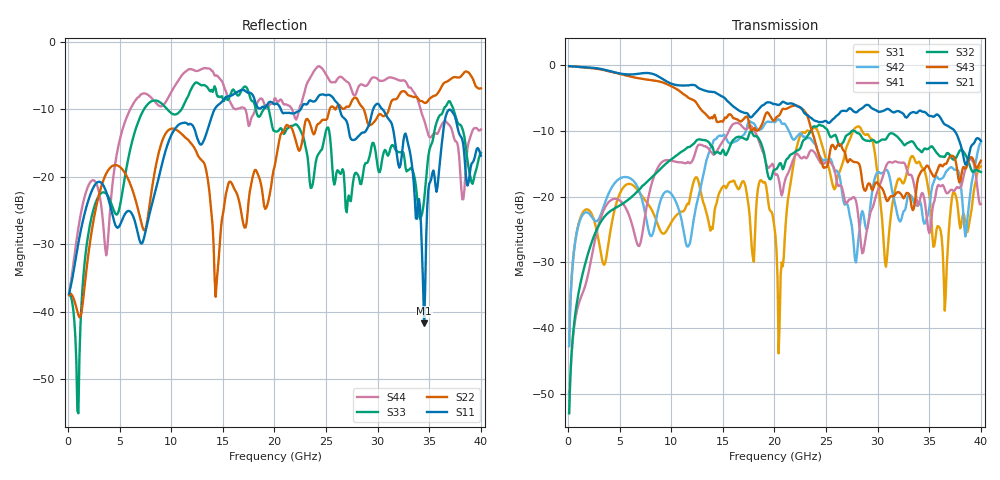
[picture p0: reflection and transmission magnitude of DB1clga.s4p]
! ADC12DJ3200QML-SP
! 196-pin ZMX package
! CLGA Ceramic Package without columns (ceramic land grid array)
! Texas Instruments 4/21/2021
! Single-ended  S-parameters
! PORT#  PORT_NAME  NET_NAME
! PORT1:  DAxN.DIEBUMP DAxN
! PORT2:  DAxN.BGA  DAxN
! PORT3:  DAxP.DIEBUMP DAxP
! PORT4:  DAxP.BGA  DAxP
! Touchstone Ver. 1.0
! Number of ports is 4
# Hz	S	MA	R	50.000000
! SCATTERING PARAMETERS  :
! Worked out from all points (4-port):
!   400 points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, 100 MHz to 40 GHz, reference 50 ohm
!   strongest paths, dB at 100 MHz, 10.1 GHz, 20.1 GHz, 30.1 GHz, 40 GHz:
!     S21: -0.1, -2.8, -5.9, -7.1, -11.5
!     S43: -0.1, -3.2, -8.1, -18.2, -14.5
!     S32: -53.0, -14.2, -15.9, -11.6, -16.2
!     S41: -52.9, -14.5, -16.7, -18.7, -21.1
!     S42: -42.7, -19.8, -8.6, -16.2, -11.7
!     S31: -42.7, -23.6, -26.1, -18.4, -15.3
!   lowest |S11| = -41.7 dB at 34.5 GHz (marker M1), VSWR 1.02, Z = 50.7 + j0.457 ohm
!   |S11| at or under -10 dB: start of sweep to 14.2 GHz; 26.32 GHz to 29.57 GHz (3.243 GHz wide, 11.6 % of centre); 30.45 GHz to end of sweep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
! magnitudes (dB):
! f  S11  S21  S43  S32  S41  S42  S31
! 100 MHz  -37.3  -0.1  -0.1  -53.0  -52.9  -42.7  -42.7
! 4 GHz  -23.8  -0.9  -0.9  -22.3  -20.7  -19.3  -26.2
! 19.1 GHz  -9.8  -5.8  -7.6  -14.3  -14.4  -8.8  -17.8
! 20.4 GHz  -9.4  -6.0  -7.7  -15.2  -17.2  -8.2  -43.8
! 25.3 GHz  -7.9  -8.8  -13.9  -10.6  -14.6  -14.3  -15.8
! 34.5 GHz  -41.7  -7.1  -15.9  -12.7  -20.2  -24.1  -15.9
! 40 GHz  -16.9  -11.5  -14.5  -16.2  -21.1  -11.7  -15.3
